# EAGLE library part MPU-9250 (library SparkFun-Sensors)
MPU-9250 9 Degree of Freedom IMU System in Package that contains MPU-6500 & AK8963 NC pin 19. 2-6 & 14-17 not internally connected. May be used for PCB trace routing. Datasheet SparkFun Products: SparkFun 9DoF Razor IMU M0 SparkFun IMU Breakout - MPU-9250
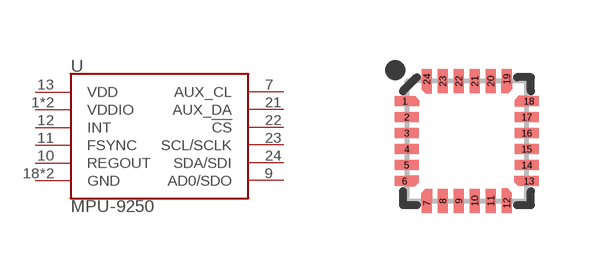
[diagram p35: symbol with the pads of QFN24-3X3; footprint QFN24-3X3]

Designator prefix U

## MPU-9250 (PROD_ID: IC-13192; VALUE: 9DoF IMU)  [QFN24-3X3]
1  VDDIO
7  AUX_CL
8  VDDIO
9  AD0/SDO
10  REGOUT
11  FSYNC
12  INT
13  VDD
18  GND
20  GND
21  AUX_DA
22  !CS
23  SCL/SCLK
24  SDA/SDI

## Footprint QFN24-3X3 (pad centres in mm)
24-Pin QFN - 3.0 x 3.0 mm - No center pad Note: No center pad per "Exposed Die Pad Precautions" section of the InvenSense MEMS Handling application note.
smd 0.495 x 0.25: 1 -1.552,1; 6 -1.552,-1; 13 1.552,-1; 18 1.552,1
smd 0.6 x 0.25: 2 -1.5,0.6; 3 -1.5,0.2; 4 -1.5,-0.2; 5 -1.5,-0.6; 14 1.5,-0.6; 15 1.5,-0.2; 16 1.5,0.2; 17 1.5,0.6
smd 0.25 x 0.495: 7 -1,-1.552; 12 1,-1.552; 19 1,1.552; 24 -1,1.552
smd 0.25 x 0.6: 8 -0.6,-1.5; 9 -0.2,-1.5; 10 0.2,-1.5; 11 0.6,-1.5; 20 0.6,1.5; 21 0.2,1.5; 22 -0.2,1.5; 23 -0.6,1.5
